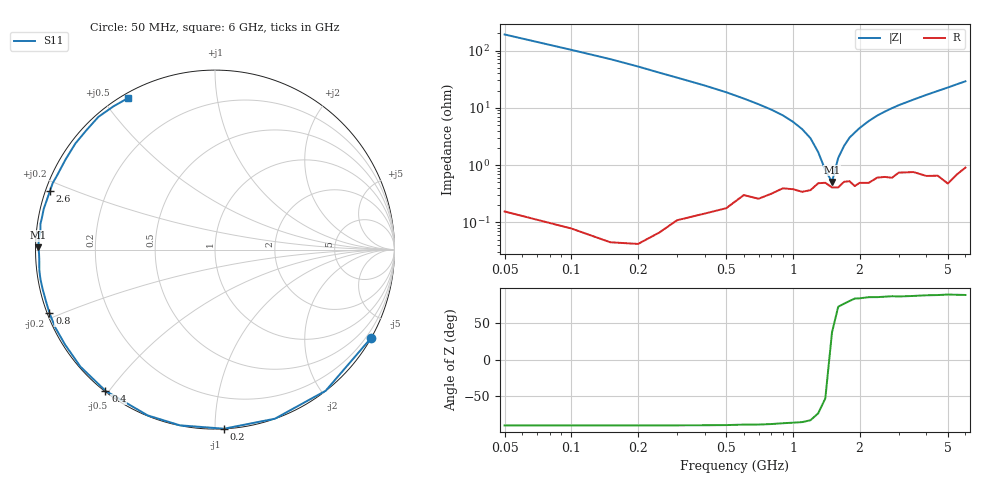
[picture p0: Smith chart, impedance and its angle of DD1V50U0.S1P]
! Infineon Technologies  Discrete & RF Semiconductors
! BBY58-02W
! Si Tuning Diode in SCD-80
! VR = 1.5 V
! S-Parameters:  June  2000
# GHz  S  MA  R  50
!  f  S11
! GHz  MAG  ANG
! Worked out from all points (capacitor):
!   34 points, 50 MHz to 6 GHz, reference 50 ohm
!   read as one part to ground: C = 15.4 pF near 50 MHz
!   lowest |Z| = 510 mohm at 1.5 GHz (marker M1)
!   series resonance near 1.468 GHz, so ESL is about 760 pH
!   S11 on the Smith chart (normalised r, x): 50 MHz: 0.00, -3.81; 200 MHz: 0.00, -1.05; 400 MHz: 0.00, -0.49; 800 MHz: 0.01, -0.19; 2.6 GHz: 0.01, +0.17; 6 GHz: 0.02, +0.58
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0.05  0.9996 -29.4
0.1  0.9994 -51.9
0.15  0.9994 -70.5
0.2  0.9992 -87.1
0.25  0.9984 -101.3
0.3  0.997 -112.1
0.4  0.9954 -127.8
0.5  0.9938 -139.0
0.6  0.989 -147.6
0.7  0.9902 -154.0
0.8  0.9878 -159.0
1  0.9851 -167.0
1.1  0.9865 -170.3
1.3  0.9809 -176.3
1.5  0.9838 179.3
1.6  0.9838 177.1
1.8  0.9793 173.2
1.9  0.983 171.6
2.2  0.9808 166.6
2.4  0.9766 163.4
2.6  0.9761 160.5
2.8  0.9771 157.7
3  0.9722 155.0
3.5  0.9723 148.9
4  0.977 142.8
5  0.9843 131.3
5.5  0.9784 125.4
6  0.9733 119.7
